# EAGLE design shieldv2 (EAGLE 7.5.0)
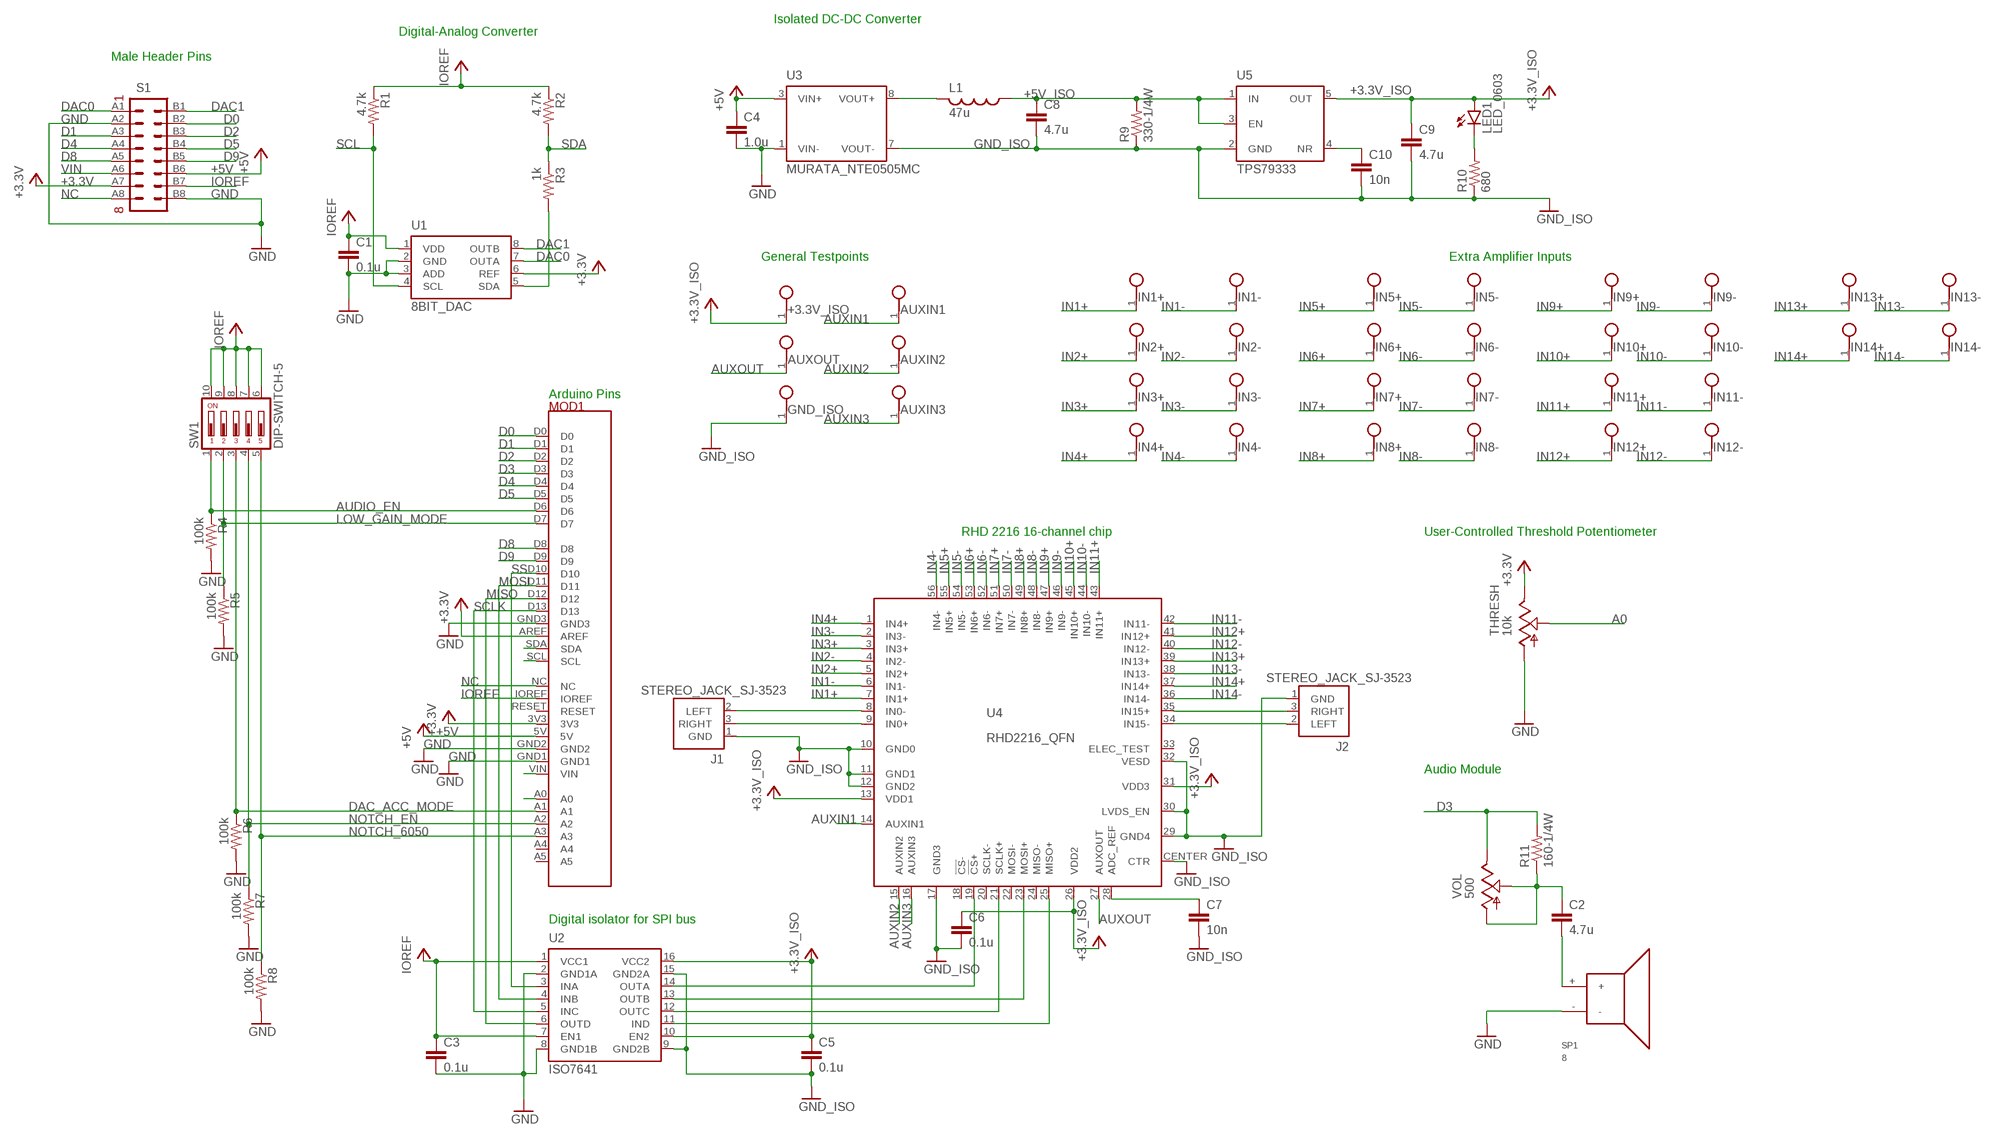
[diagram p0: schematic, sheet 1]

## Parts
+3.3V_ISO  TESTPOINT  [TESTPOINT]
AUXIN1  TESTPOINT  [TESTPOINT]
AUXIN2  TESTPOINT  [TESTPOINT]
AUXIN3  TESTPOINT  [TESTPOINT]
AUXOUT  TESTPOINT  [TESTPOINT]
C1  0.1u  C_0603  [0603]
C2  4.7u  C_0805  [0805]
C3  0.1u  C_0603  [0603]
C4  1.0u  C_0805  [0805]
C5  0.1u  C_0603  [0603]
C6  0.1u  C_0603  [0603]
C7  10n  C_0603  [0603]
C8  4.7u  C_0805  [0805]
C9  4.7u  C_0805  [0805]
C10  10n  C_0603  [0603]
GND_ISO  TESTPOINT  [TESTPOINT]
IN1+  TESTPOINT  [TESTPOINT]
IN1-  TESTPOINT  [TESTPOINT]
IN2+  TESTPOINT  [TESTPOINT]
IN2-  TESTPOINT  [TESTPOINT]
IN3+  TESTPOINT  [TESTPOINT]
IN3-  TESTPOINT  [TESTPOINT]
IN4+  TESTPOINT  [TESTPOINT]
IN4-  TESTPOINT  [TESTPOINT]
IN5+  TESTPOINT  [TESTPOINT]
IN5-  TESTPOINT  [TESTPOINT]
IN6+  TESTPOINT  [TESTPOINT]
IN6-  TESTPOINT  [TESTPOINT]
IN7+  TESTPOINT  [TESTPOINT]
IN7-  TESTPOINT  [TESTPOINT]
IN8+  TESTPOINT  [TESTPOINT]
IN8-  TESTPOINT  [TESTPOINT]
IN9+  TESTPOINT  [TESTPOINT]
IN9-  TESTPOINT  [TESTPOINT]
IN10+  TESTPOINT  [TESTPOINT]
IN10-  TESTPOINT  [TESTPOINT]
IN11+  TESTPOINT  [TESTPOINT]
IN11-  TESTPOINT  [TESTPOINT]
IN12+  TESTPOINT  [TESTPOINT]
IN12-  TESTPOINT  [TESTPOINT]
IN13+  TESTPOINT  [TESTPOINT]
IN13-  TESTPOINT  [TESTPOINT]
IN14+  TESTPOINT  [TESTPOINT]
IN14-  TESTPOINT  [TESTPOINT]
J1  STEREO_JACK_SJ-3523  [SJ-3523]
J2  STEREO_JACK_SJ-3523  [SJ-3523]
L1  47u  L_1210  [1210]
LED1  LED_0603  [0603_DIODE]
MOD1  UNOHEADERS  [UNOHEADERS]
R1  4.7k  R_0603  [0603]
R2  4.7k  R_0603  [0603]
R3  1k  R_0603  [0603]
R4  100k  R_0603  [0603]
R5  100k  R_0603  [0603]
R6  100k  R_0603  [0603]
R7  100k  R_0603  [0603]
R8  100k  R_0603  [0603]
R9  330-1/4W  R_0603  [0603]
R10  680  R_0603  [0603]
R11  160-1/4W  R_0603  [0603]
S1  100MIL_HEADER_8X2  [100MIL_HEADER_8X2]
SP1  8  PCM_SPEAKER  [PCM_SPEAKER]
SW1  DIP-SWITCH-5  [DIP-SWITCH-5]
THRESH  10k  POT_SLIDE  [SLIDE_POT_REPLACEMENT]
U1  8BIT_DAC  [UMAX]
U2  ISO7641  [SOIC-16-WIDE]
U3  MURATA_NTE0505MC  [MURATA_NTE]
U4  RHD2216_QFN  [QFN56_8_X_8_LARGE]
U5  TPS79333  [SOT-23-5]
VOL  500  POT_ROT  [ROT_POT_REPLACEMENT]

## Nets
+3.3V: MOD1.3V3 MOD1.AREF S1.A7 THRESH.3 U1.6(REF)
+3.3V_ISO [power]: +3.3V_ISO.1 C5.1 C6.1 C9.1 LED1.A U2.10(EN2) U2.16(VCC2) U4.13(VDD1) U4.26(VDD2) U4.31(VDD3) U5.5(OUT)
+5V: C4.1 MOD1.5V S1.B6 U3.3(VIN+)
+5V_ISO [power]: C8.1 L1.1 R9.2 U5.1(IN) U5.3(EN)
A0: MOD1.A0 THRESH.2
AUDIO_EN: MOD1.D6 R4.1 SW1.1
AUXIN1: AUXIN1.1 U4.14(AUXIN1)
AUXIN2: AUXIN2.1 U4.15(AUXIN2)
AUXIN3: AUXIN3.1 U4.16(AUXIN3)
AUXOUT: AUXOUT.1 U4.27(AUXOUT)
D0: MOD1.D0 S1.B2
D1: MOD1.D1 S1.A3
D2: MOD1.D2 S1.B3
D3: MOD1.D3 R11.2 VOL.3
D4: MOD1.D4 S1.A4
D5: MOD1.D5 S1.B4
D8: MOD1.D8 S1.A5
D9: MOD1.D9 S1.B5
DAC0: S1.A1 U1.7(OUTA)
DAC1: S1.B1 U1.8(OUTB)
DAC_ACC_MODE: MOD1.A1 R6.1 SW1.3
GND: C1.2 C3.2 C4.2 MOD1.GND1 MOD1.GND2 MOD1.GND3 R4.2 R5.2 R6.2 R7.2 R8.2 S1.A2 S1.B8 SP1.- THRESH.1 U1.2(GND) U1.3(ADD) U2.2(GND1A) U2.8(GND1B) U3.1(VIN-)
GND_ISO: C5.2 C6.2 C7.2 C8.2 C9.2 C10.2 GND_ISO.1 J1.1(GND) J2.1(GND) R9.1 R10.1 U2.9(GND2B) U2.15(GND2A) U3.7(VOUT-) U4.10(GND0) U4.11(GND1) U4.12(GND2) U4.17(GND3) U4.29(GND4) U4.30(LVDS_EN) U4.32(VESD) U4.CENTER(CTR) U5.2(GND)
IN1+ [power]: IN1+.1 U4.7(IN1+)
IN1-: IN1-.1 U4.6(IN1-)
IN2+: IN2+.1 U4.5(IN2+)
IN2-: IN2-.1 U4.4(IN2-)
IN3+: IN3+.1 U4.3(IN3+)
IN3-: IN3-.1 U4.2(IN3-)
IN4+: IN4+.1 U4.1(IN4+)
IN4-: IN4-.1 U4.56(IN4-)
IN5+ [power]: IN5+.1 U4.55(IN5+)
IN5-: IN5-.1 U4.54(IN5-)
IN6+ [power]: IN6+.1 U4.53(IN6+)
IN6-: IN6-.1 U4.52(IN6-)
IN7+: IN7+.1 U4.51(IN7+)
IN7-: IN7-.1 U4.50(IN7-)
IN8+: IN8+.1 U4.49(IN8+)
IN8-: IN8-.1 U4.48(IN8-)
IN9+: IN9+.1 U4.47(IN9+)
IN9-: IN9-.1 U4.46(IN9-)
IN10+ [power]: IN10+.1 U4.45(IN10+)
IN10-: IN10-.1 U4.44(IN10-)
IN11+: IN11+.1 U4.43(IN11+)
IN11-: IN11-.1 U4.42(IN11-)
IN12+: IN12+.1 U4.41(IN12+)
IN12-: IN12-.1 U4.40(IN12-)
IN13+: IN13+.1 U4.39(IN13+)
IN13-: IN13-.1 U4.38(IN13-)
IN14+: IN14+.1 U4.37(IN14+)
IN14-: IN14-.1 U4.36(IN14-)
IOREF: C1.1 C3.1 MOD1.IOREF R1.1 R2.1 S1.B7 SW1.6 SW1.7 SW1.8 SW1.9 SW1.10 U1.1(VDD) U2.1(VCC1) U2.7(EN1)
LOW_GAIN_MODE: MOD1.D7 R5.1 SW1.2
MISO: MOD1.D12 U2.6(OUTD)
MOSI: MOD1.D11 U2.4(INB)
N$1: U2.14(OUTA) U4.19(!CS!+)
N$2: C2.1 R11.1 VOL.1 VOL.2
N$3: C2.2 SP1.+
N$4: U2.13(OUTB) U4.23(MOSI+)
N$6: U2.12(OUTC) U4.21(SCLK+)
N$7: U2.11(IND) U4.25(MISO+)
N$11: L1.2 U3.8(VOUT+)
N$12: LED1.C R10.2
N$13: C7.1 U4.28(ADC_REF)
N$14: C10.1 U5.4(NR)
N$18: J1.2(LEFT) U4.8(IN0-)
N$19: J1.3(RIGHT) U4.9(IN0+)
N$30: J2.3(RIGHT) U4.35(IN15+)
N$31: J2.2(LEFT) U4.34(IN15-)
NC: MOD1.NC S1.A8
NOTCH_6050: MOD1.A3 R8.1 SW1.5
NOTCH_EN: MOD1.A2 R7.1 SW1.4
PRESDA: R3.2 U1.5(SDA)
SCL: MOD1.SCL R1.2 U1.4(SCL)
SCLK: MOD1.D13 U2.5(INC)
SDA: MOD1.SDA R2.2 R3.1
SS: MOD1.D10 U2.3(INA)
VIN: MOD1.VIN S1.A6
Unconnected: MOD1.A4 MOD1.A5 MOD1.RESET U4.18(!CS!-) U4.20(SCLK-) U4.22(MOSI-) U4.24(MISO-) U4.33(ELEC_TEST)

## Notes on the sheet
- Isolated DC-DC Converter
- Digital-Analog Converter
- Male Header Pins
- General Testpoints | Extra Amplifier Inputs
- Arduino Pins
- RHD 2216 16-channel chip | User-Controlled Threshold Potentiometer
- Audio Module
- Digital isolator for SPI bus

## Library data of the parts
+3.3V_ISO AUXIN1-AUXIN3 AUXOUT GND_ISO IN1+ IN1- IN2+ IN2- IN3+ IN3- IN4+ IN4- IN5+ IN5- IN6+ IN6- IN7+ IN7- IN8+ IN8- IN9+ IN9- IN10+ IN10- IN11+ IN11- IN12+ IN12- IN13+ IN13- IN14+ IN14- = RHD2000_eval_board:TESTPOINT: PCB Test Point
C1-C10 = CLAMP_interface_board:C: Capacitor
J1 J2 = CLAMP_interface_board:STEREO_JACK: CUI Inc. SJ-3523 stereo audio jack
L1 = CLAMP_interface_board:L: Inductor
LED1 = CLAMP_interface_board:LED
MOD1 = intan-arduino:UNOHEADERS: Headers for connecting an Arduino UNO to a shield
R1-R11 = CLAMP_interface_board:R: Resistor
S1 = intan-arduino:100MIL_HEADER_8X2: 8 rows of 2 header pins, 100 mil spacing. DigiKey: 609-3486-1-ND
SP1 = intan-arduino:PCM_SPEAKER
SW1 = intan-arduino:DIP-SWITCH-5
THRESH VOL = intan-arduinov2:POT: Potentiometer
U1 = intan-arduino:8BIT_DAC: 8-bit 2 Wire Serial DAC. Digikey Part Number MAX5820LEUA+-ND
U2 = CLAMP_interface_board:ISO7641: TI ISO7641FM Quad-Channel Digital Isolator
U3 = CLAMP_interface_board:MURATA_NTE0505MC: Murata NTE0505MC Isolated 1W +5V to +5V DC/DC Converter
U4 = harrison:RHD2216
U5 = CLAMP_interface_board:TPS79333: Texas Instruments TPS79333 3.3V LDO regulator

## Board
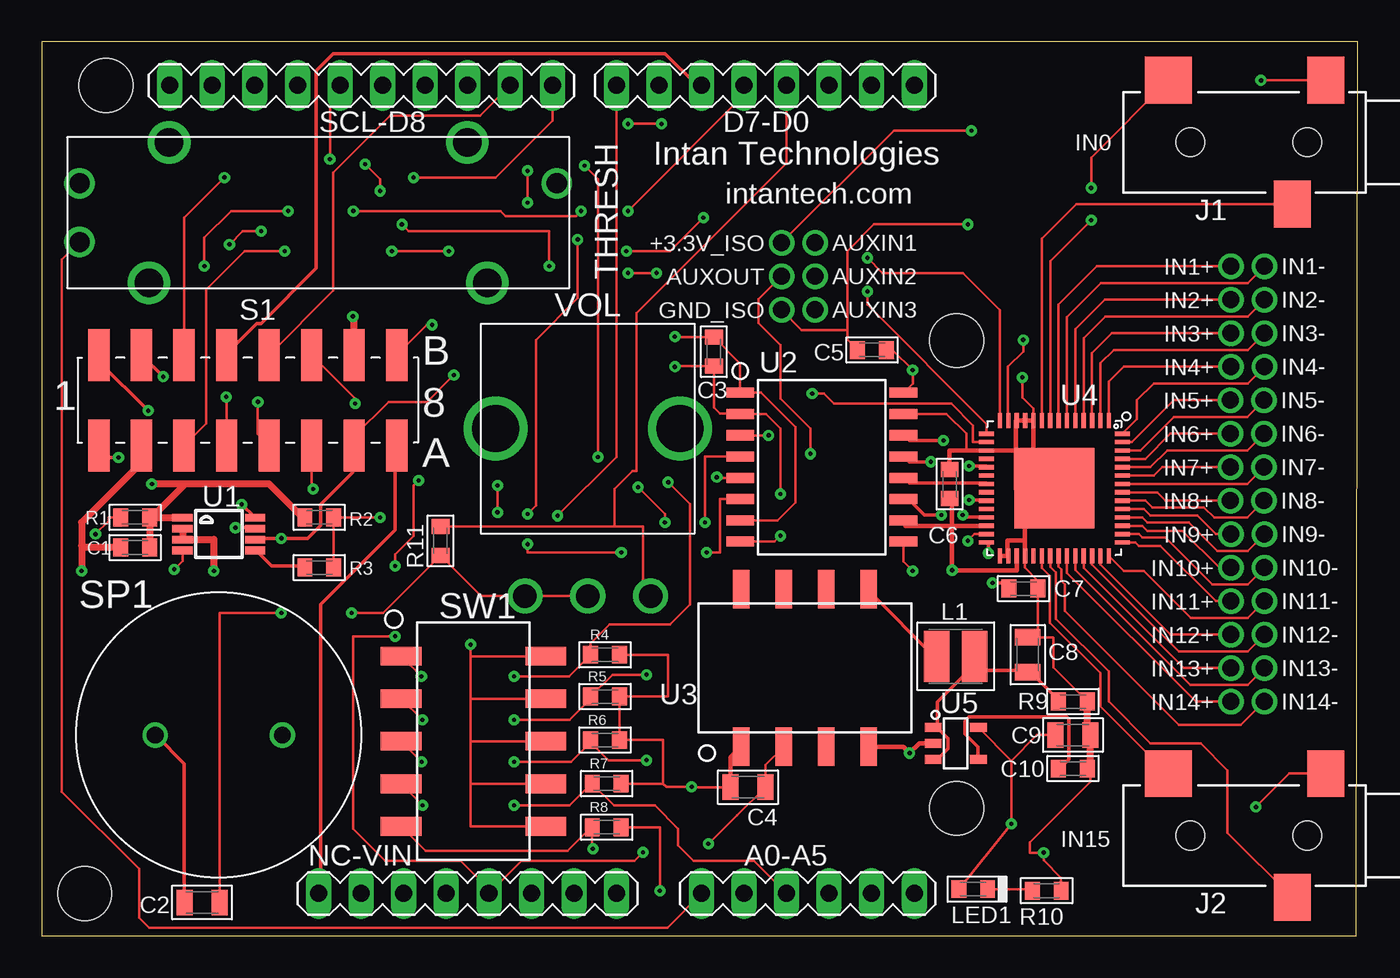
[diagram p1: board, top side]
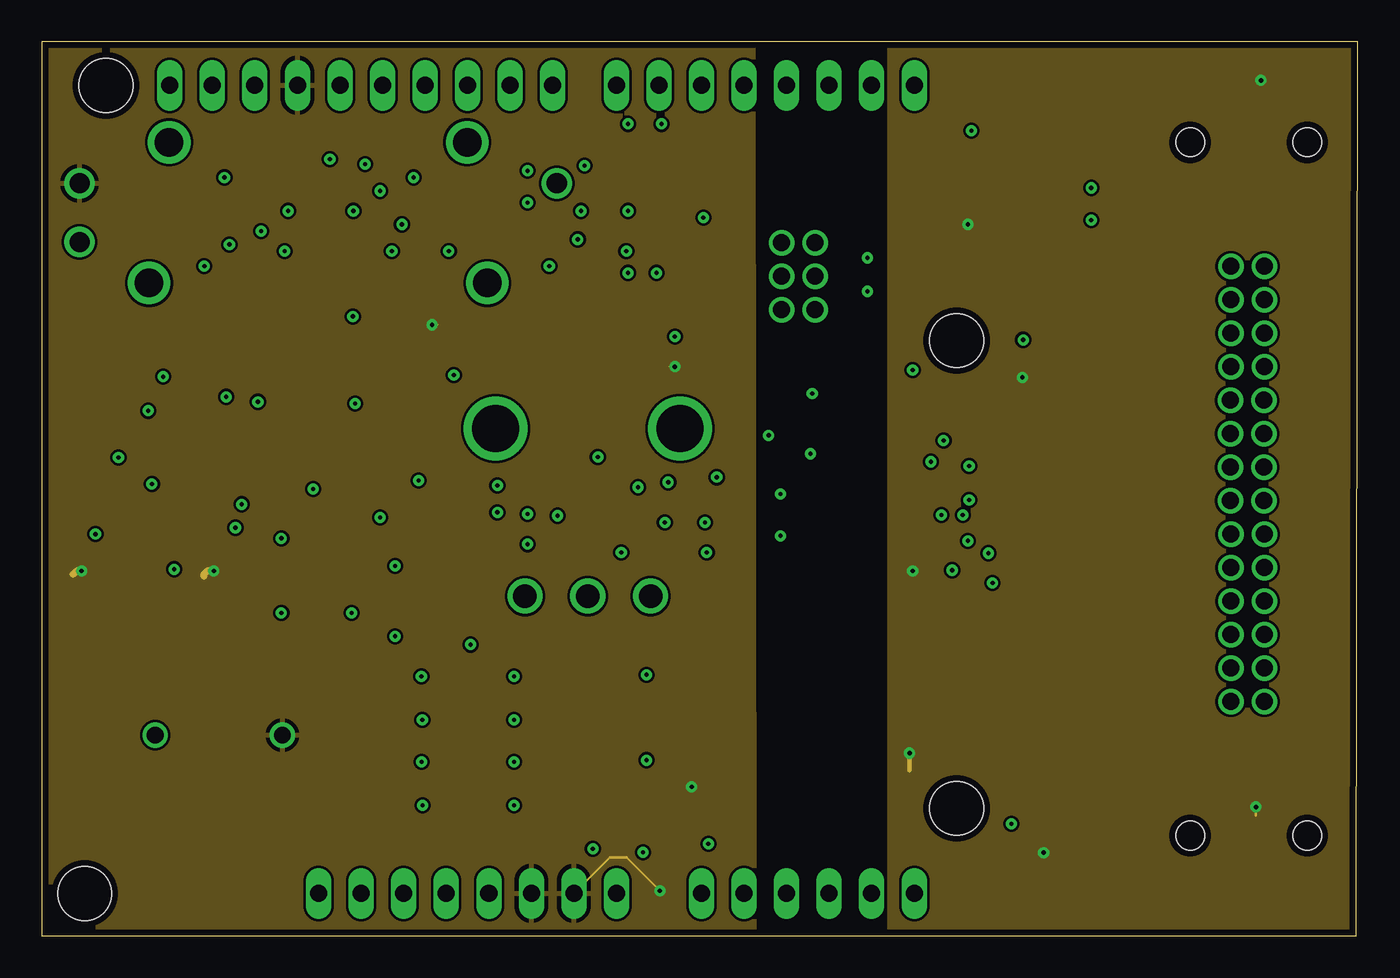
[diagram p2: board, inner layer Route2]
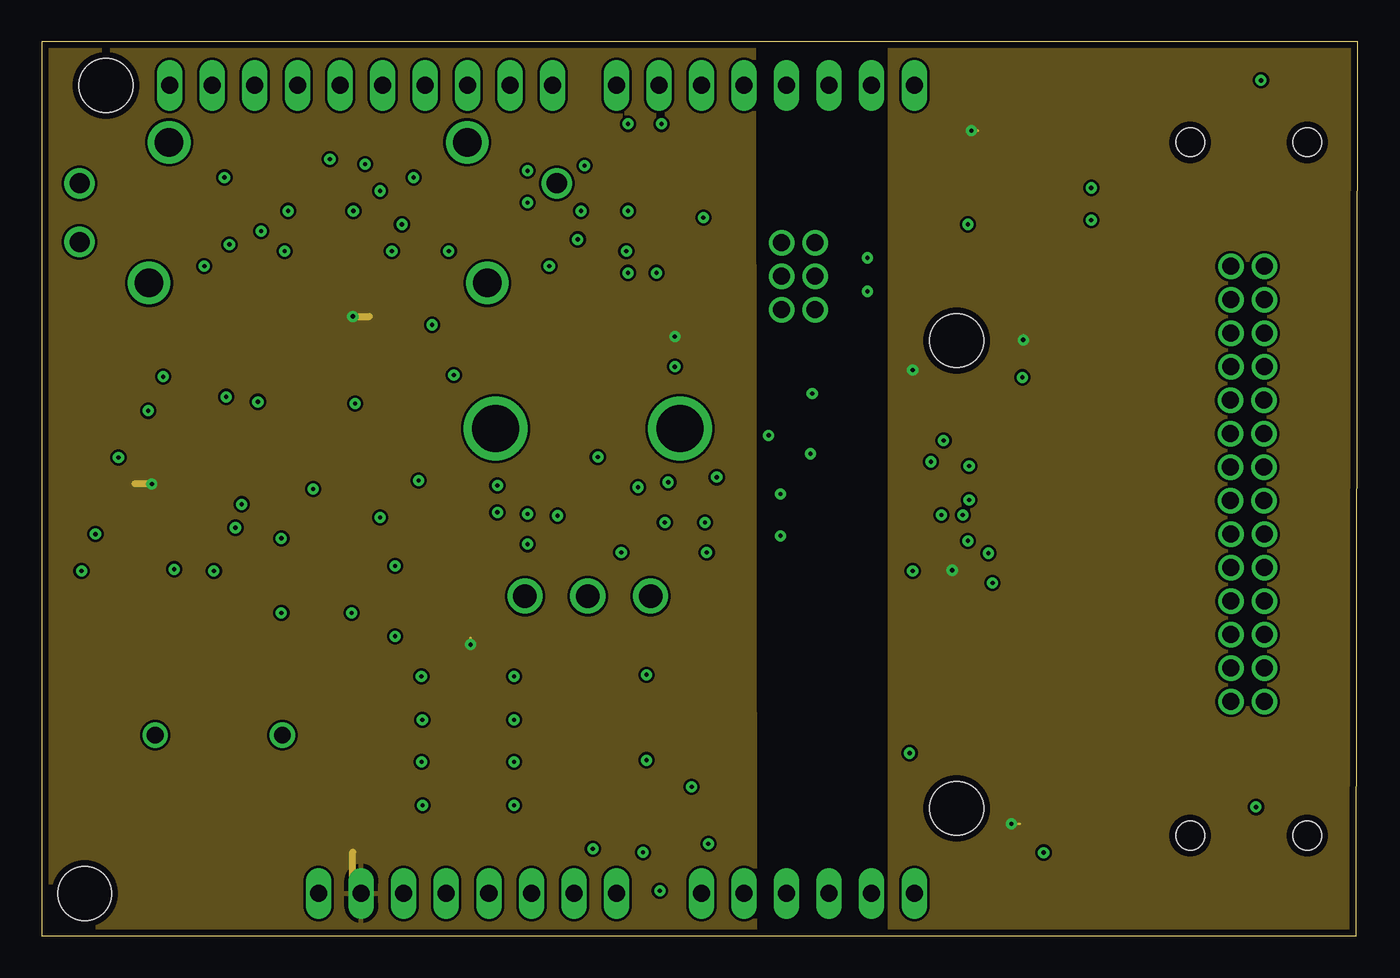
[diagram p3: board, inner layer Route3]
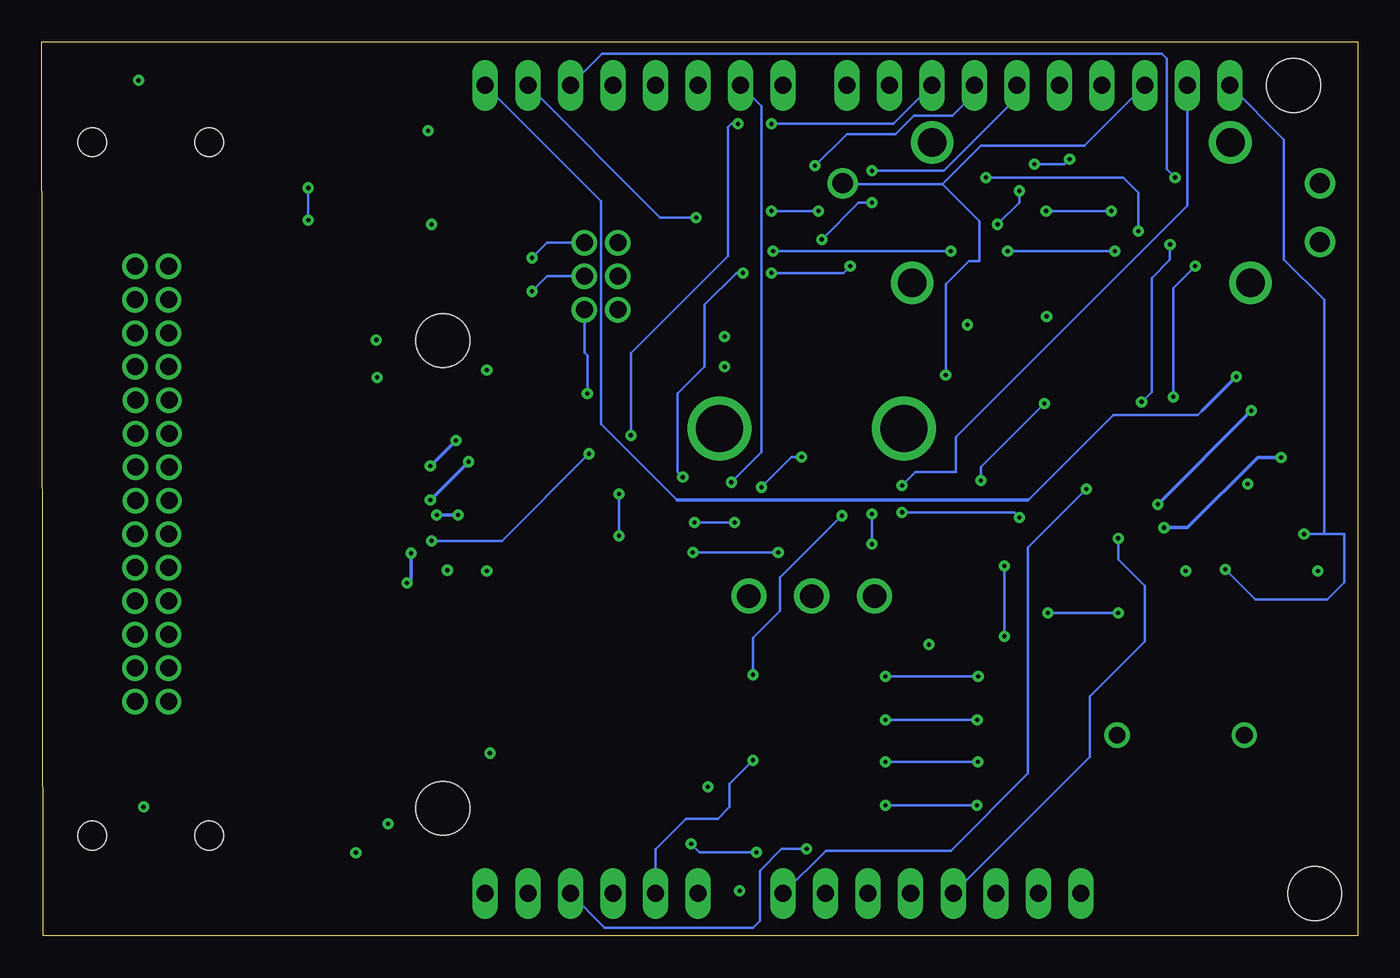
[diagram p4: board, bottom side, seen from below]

Size 78.57 x 53.4 mm. Coordinates in mm from the lower left corner, seen from the top.
Outline: 0,0 78.5,0 78.57,53.4 0,53.4 0,0
Copper layers (1*2+3*16): Top 0.035mm / dielectric 1.5mm / Route2 0.035mm / dielectric 0.15mm / Route3 0.035mm / dielectric 0.2mm / Bottom 0.035mm
Design rules "default *": minimum track width 6mil, minimum drill 10mil, track to track 6mil, track to pad 6mil, pad to pad 6mil, via to via 6mil, smd to smd 6mil, copper to edge 15mil, drill to drill 8mil, minimum pad ring 10mil, minimum via ring 8mil, stop-mask expansion 4mil, vias tented up to drill 0mil, thermal gap 10mil

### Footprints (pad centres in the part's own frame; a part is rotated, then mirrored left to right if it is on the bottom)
TESTPOINT = drill 1.016: 1 0,0
0603 = smd 0.889 x 1.067: 1 -0.864,0; 2 0.864,0
0805 = smd 0.965 x 1.524: 1 -1.041,0; 2 1.041,0
SJ-3523 = smd 2.2 x 2.8: 1 -1.1,-3.7; 3 0.9,3.7 | smd 2.8 x 2.8: 2 8.3,-3.7 | hole 1.7: 7,0; 0,0
1210 = smd 1.524 x 3.048: 1 -1.143,0; 2 1.143,0
0603_DIODE = smd 0.889 x 1.067: A 0.864,0; C -0.864,0
UNOHEADERS = drill 1.016 long: 3V3 -29.21,-49.53; 5V -26.67,-49.53; A0 -13.97,-49.53; A1 -11.43,-49.53; A2 -8.89,-49.53; A3 -6.35,-49.53; A4 -3.81,-49.53; A5 -1.27,-49.53; AREF -40.64,-1.27; D0 -1.27,-1.27; D1 -3.81,-1.27; D2 -6.35,-1.27; D3 -8.89,-1.27; D4 -11.43,-1.27; D5 -13.97,-1.27; D6 -16.51,-1.27; D7 -19.05,-1.27; D8 -22.86,-1.27; D9 -25.4,-1.27; D10 -27.94,-1.27; D11 -30.48,-1.27; D12 -33.02,-1.27; D13 -35.56,-1.27; GND1 -21.59,-49.53; GND2 -24.13,-49.53; GND3 -38.1,-1.27; IOREF -34.29,-49.53; NC -36.83,-49.53; RESET -31.75,-49.53; SCL -45.72,-1.27; SDA -43.18,-1.27; VIN -19.05,-49.53 | hole 3.2: -49.53,-1.27; 1.27,-16.51; 1.27,-44.45; -50.8,-49.53
100MIL_HEADER_8X2 = smd 1.27 x 3.1: A1 -10.16,-2.7; A2 -7.62,-2.7; A3 -5.08,-2.7; A4 -2.54,-2.7; A5 0,-2.7; A6 2.54,-2.7; A7 5.08,-2.7; A8 7.62,-2.7; B1 -10.16,2.7; B2 -7.62,2.7; B3 -5.08,2.7; B4 -2.54,2.7; B5 0,2.7; B6 2.54,2.7; B7 5.08,2.7; B8 7.62,2.7
PCM_SPEAKER = drill 1: + -3.8,0; - 3.8,0
DIP-SWITCH-5 = smd 1.118 x 2.438: 1 -3.81,-4.318; 2 -1.27,-4.318; 3 1.27,-4.318; 4 3.81,-4.318; 5 6.35,-4.318; 6 6.35,4.318; 7 3.81,4.318; 8 1.27,4.318; 9 -1.27,4.318; 10 -3.81,4.318
SLIDE_POT_REPLACEMENT = drill 1.2: 1 -14.25,1.75; 2 -14.25,-1.75; 3 14.25,1.75 | drill 1.7: H1 -10.1,-4.2; H2 10.1,-4.2; H3 8.9,4.2; H4 -8.9,4.2
UMAX = smd 0.45 x 1.2: 1 -0.975,-2.175; 2 -0.325,-2.175; 3 0.325,-2.175; 4 0.975,-2.175; 5 0.975,2.175; 6 0.325,2.175; 7 -0.325,2.175; 8 -0.975,2.175
SOIC-16-WIDE = smd 0.6 x 1.65: 1 -4.445,-4.875; 2 -3.175,-4.875; 3 -1.905,-4.875; 4 -0.635,-4.875; 5 0.635,-4.875; 6 1.905,-4.875; 7 3.175,-4.875; 8 4.445,-4.875; 9 4.445,4.875; 10 3.175,4.875; 11 1.905,4.875; 12 0.635,4.875; 13 -0.635,4.875; 14 -1.905,4.875; 15 -3.175,4.875; 16 -4.445,4.875
MURATA_NTE = smd 1 x 2.3: 1 -3.81,-4.7; 3 -1.27,-4.7; 5 1.27,-4.7; 7 3.81,-4.7; 8 3.81,4.7; 10 1.27,4.7; 12 -1.27,4.7; 14 -3.81,4.7
QFN56_8_X_8_LARGE = smd 0.9 x 0.25: 1 -4.05,3.25; 2 -4.05,2.75; 3 -4.05,2.25; 4 -4.05,1.75; 5 -4.05,1.25; 6 -4.05,0.75; 7 -4.05,0.25; 8 -4.05,-0.25; 9 -4.05,-0.75; 10 -4.05,-1.25; 11 -4.05,-1.75; 12 -4.05,-2.25; 13 -4.05,-2.75; 14 -4.05,-3.25; 29 4.05,-3.25; 30 4.05,-2.75; 31 4.05,-2.25; 32 4.05,-1.75; 33 4.05,-1.25; 34 4.05,-0.75; 35 4.05,-0.25; 36 4.05,0.25; 37 4.05,0.75; 38 4.05,1.25; 39 4.05,1.75; 40 4.05,2.25; 41 4.05,2.75; 42 4.05,3.25 | smd 0.25 x 0.9: 15 -3.25,-4.05; 16 -2.75,-4.05; 17 -2.25,-4.05; 18 -1.75,-4.05; 19 -1.25,-4.05; 20 -0.75,-4.05; 21 -0.25,-4.05; 22 0.25,-4.05; 23 0.75,-4.05; 24 1.25,-4.05; 25 1.75,-4.05; 26 2.25,-4.05; 27 2.75,-4.05; 28 3.25,-4.05; 43 3.25,4.05; 44 2.75,4.05; 45 2.25,4.05; 46 1.75,4.05; 47 1.25,4.05; 48 0.75,4.05; 49 0.25,4.05; 50 -0.25,4.05; 51 -0.75,4.05; 52 -1.25,4.05; 53 -1.75,4.05; 54 -2.25,4.05; 55 -2.75,4.05; 56 -3.25,4.05 | smd 4.8 x 4.8: CENTER 0,0
SOT-23-5 = smd 0.55 x 1: 1 -0.95,-1.35; 2 0,-1.35; 3 0.95,-1.35; 4 0.95,1.35; 5 -0.95,1.35
ROT_POT_REPLACEMENT = drill 1.4: 1 -3.75,-10; 2 0,-10; 3 3.75,-10 | drill 2.8: H1 -5.5,0; H2 5.5,0

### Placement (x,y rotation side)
+3.3V_ISO  44.17,41.4 180 top
AUXIN1  46.17,41.4 0 top
AUXIN2  46.17,39.4 0 top
AUXIN3  46.17,37.4 0 top
AUXOUT  44.17,39.4 180 top
C1  5.57,23.2 180 top
C2  9.57,2 180 top
C3  40.13,34.9 270 top
C4  42.16,8.89 180 top
C5  49.57,35 180 top
C6  54.21,26.98 90 top
C7  58.62,20.75 0 top
C8  58.87,16.8 90 top
C9  61.57,12 0 top
C10  61.57,10 0 top
GND_ISO  44.17,37.4 180 top
IN1+  71,40 180 top
IN1-  73,40 0 top
IN2+  71,38 180 top
IN2-  73,38 0 top
IN3+  71,36 180 top
IN3-  73,36 0 top
IN4+  71,34 180 top
IN4-  73,34 0 top
IN5+  70.97,32 180 top
IN5-  72.97,32 0 top
IN6+  70.97,30 180 top
IN6-  72.97,30 0 top
IN7+  70.97,28 180 top
IN7-  72.97,28 0 top
IN8+  70.97,26 180 top
IN8-  72.97,26 0 top
IN9+  71,24 180 top
IN9-  73,24 0 top
IN10+  71,22 180 top
IN10-  73,22 0 top
IN11+  71,20 180 top
IN11-  73,20 0 top
IN12+  71,18 180 top
IN12-  73,18 0 top
IN13+  71,16 180 top
IN13-  73,16 0 top
IN14+  71,14 180 top
IN14-  73,14 0 top
J1  75.57,47.4 180 top
J2  75.57,6 180 top
L1  54.57,16.7 180 top
LED1  55.61,2.8 180 top
MOD1  53.36,52.07 0 top
R1  5.57,25 180 top
R2  16.57,25 0 top
R3  16.57,22 180 top
R4  33.63,16.8 0 top
R5  33.63,14.3 0 top
R6  33.63,11.7 0 top
R7  33.73,9.1 0 top
R8  33.73,6.5 0 top
R9  61.57,14 180 top
R10  60,2.7 180 top
R11  23.8,23.6 90 top
S1  13.57,32 0 top
SP1  10.57,12 0 top
SW1  25.77,12.9 270 top
THRESH  16.5,43.2 0 top
U1  10.57,24 270 top
U2  46.57,28 270 top
U3  45.57,16 0 top
U4  60.46,26.75 270 top
U5  54.57,11.5 270 top
VOL  32.6,30.3 0 top

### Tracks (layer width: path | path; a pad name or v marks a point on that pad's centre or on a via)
+3.3V  (via drill 0.25)
  Top 0.152: v24.6,33.5 23,31.9 20.7,31.9 18.65,29.85 S1.A7
  Top 0.203: U1.6 12.83,23.75 v14.3,23.75 15.88,23.75 16.64,24.51 16.64,25.78 18.54,27.69 18.54,29.21 S1.A7
  Bottom 0.152: v24.6,33.5 24.6,38.92 23.22,40.3 22.6,40.3 22.6,42.7 24.8,44.9 | MOD1.3V3 16,10.69 16,14.3 12.7,17.6 12.7,20.9 14.3,22.5 v14.3,23.75 | MOD1.AREF 16.32,47.2 22.5,47.2 24.8,44.9 | 24.8,44.9 30.7,44.9 THRESH.3
+3.3V_ISO  (via drill 0.25)
  Top 0.152: U5.5 57.9,10.47 | 57.9,10.47 v57.9,6.7 LED1.A | 57.9,10.47 59.43,12 C9.1 | +3.3V_ISO.1 50.87,48.1 v55.5,48.1 | U4.13 57.7,34 58.6,34.9 v58.6,35.6 | C5.1 50.8,35 v52,33.8 52,33 U2.16
  Top 0.254: U4.31 58.21,21.84 v54.36,21.84 54.36,24.5 | U2.10 51.45,24.89 51.56,24.89 51.56,24.5 54.36,24.5 | U4.26 54.36,24.5 | 54.36,24.5 54.36,25.97 C6.1
  Route3 0.152: v57.9,6.7 58.4,6.7 | v55.5,48.1 55.9,48.1 | v58.6,35.6 58.6,35.9 | v52,33.8 52.2,33.8
  pour Route3: 50.65,0 78.5,0 78.5,53.5 50.65,53.5
+5V  (via drill 0.25)
  Top 0.152: v35.9,5 35.4,4.5 28.65,4.5 MOD1.5V 26.69,2.81 25,4.5 20.5,4.5 18.6,6.4 18.6,17.9 v21.1,17.9 | v39.8,5.5 41.5,7.2 41.52,7.2 C4.1 43.2,10.21 U3.3 | S1.B6 18.7,32.11 v18.7,31.8 | v22.5,27.2 22.2,26.9 22.2,23.9 21.1,22.8 v21.1,22.1
  Bottom 0.152: v35.9,5 39.3,5 v39.8,5.5 | v18.7,31.8 22.5,28 v22.5,27.2 | v21.1,22.1 v21.1,17.9
+5V_ISO
  Top 0.203: R9.2 60.71,14.1 58.93,15.88 C8.1 58.8,15.88 55.5,15.88 L1.1 55.63,16.64 55.63,16.13 53.47,13.97 53.47,12.57 U5.1 53.34,12.57 54.1,11.81 54.1,11.18 53.59,10.67 53.34,10.67 U5.3
A0
  Top 0.152: THRESH.2 1.2,40.4 1.2,8.6 5.8,4 5.8,1.1 6.4,0.5 37.35,0.5 MOD1.A0
AUDIO_EN  (via drill 0.25)
  Top 0.152: SW1.1 v22.66,15.5 | v28.2,15.5 31.47,15.5 R4.1 32.77,17.47 33.9,18.6 37.5,18.6 38.7,19.8 38.7,25.8 v37.4,27.1
  Bottom 0.152: v28.2,15.5 v22.66,15.5 | v37.4,27.1 35.6,28.9 35.6,49.55 MOD1.D6
AUXIN1  (via drill 0.25)
  Top 0.152: U4.14 57.21,37.39 55,39.6 50.2,39.6 v49.3,40.5
  Bottom 0.152: AUXIN1.1 48.4,41.4 v49.3,40.5
AUXIN2  (via drill 0.25)
  Top 0.152: U4.15 56.41,30.59 49.3,37.7 v49.3,38.5
  Bottom 0.152: AUXIN2.1 48.4,39.4 v49.3,38.5
AUXIN3  (via drill 0.25)
  Top 0.152: U4.16 55.6,29.5 55.6,30.5 54.3,31.8 47.3,31.8 46.7,32.4 v46,32.4
  Bottom 0.152: AUXIN3.1 46.17,34.83 46,34.66 v46,32.4
AUXOUT  (via drill 0.25)
  Top 0.152: U4.27 55.7,24 v55.3,23.6 | AUXOUT.1 42.8,38.03 42.8,36.6 44.1,35.3 44.1,32.1 45.9,30.3 v45.9,28.8
  Bottom 0.152: v55.3,23.6 51.1,23.6 v45.9,28.8
D0  (via drill 0.25)
  Top 0.203: v7.24,33.4 5.97,34.67 S1.B2
  Bottom 0.152: 9.27,31.37 9.54,31.1 14.6,31.1 19.66,26.04 19.68,26.04 | 40.64,26.04 45.17,30.57 45.17,43.88 MOD1.D0
  Bottom 0.203: 19.68,26.04 40.64,26.04 | v7.24,33.4 9.27,31.37 | 52.07,50.8 MOD1.D0
D1  (via drill 0.25)
  Top 0.152: S1.A3 9.8,30.61 9.8,38.6 12.1,40.9 v14.5,40.9 | v34.9,40.9 37.5,40.9 v39.5,42.9 | v20.9,40.9 v24.3,40.9
  Bottom 0.152: v39.5,42.9 41.65,42.9 MOD1.D1 | v14.5,40.9 v20.9,40.9 | v24.3,40.9 v34.9,40.9
D2  (via drill 0.25)
  Top 0.152: S1.B3 8.49,42.89 v10.9,45.3
  Bottom 0.152: v10.9,45.3 11.4,45.8 11.4,52.4 11.7,52.7 45.11,52.7 MOD1.D2
D3
  Top 0.152: R11.2 34.2,24.46 | 34.2,24.46 35.9,24.46 35.9,20.75 VOL.3 | MOD1.D3 44.47,46.17 35.5,37.2 35.5,27.78 35.28,27.78 34.2,26.7 34.2,24.46
D4  (via drill 0.25)
  Top 0.152: S1.A4 11.03,32.17 v11,32.2 | v9.7,40 9.7,41.7 11.3,43.3 v14.7,43.3 | v35,43.3 41.93,50.23 MOD1.D4 | v32.2,43.3 31.9,43 27.7,43 27.4,43.3 v18.6,43.3
  Bottom 0.152: v11,32.2 11,38.7 v9.7,40 | v14.7,43.3 v18.6,43.3 | v32.2,43.3 v35,43.3
D5
  Top 0.203: MOD1.D5 39.12,50.8 37.21,52.7 17.4,52.7 16.38,51.69 16.38,39.88 13.08,36.58 12.83,36.58 11.05,34.8 S1.B4
D8  (via drill 0.25)
  Top 0.152: S1.A5 12.9,29.97 v12.9,31.9 | v11.2,41.3 12,42.1 v13.1,42.1 | v22.2,45.3 27.1,45.3 30.5,48.7 MOD1.D8
  Bottom 0.152: v12.9,31.9 12.3,32.5 12.3,39.3 11.2,40.4 v11.2,41.3 | v13.1,42.1 13.1,44.4 14,45.3 v22.2,45.3
D9
  Top 0.152: S1.B5 17.4,38.53 17.4,45.6 20.8,49 26.16,49 MOD1.D9
DAC0  (via drill 0.25)
  Top 0.203: v11.56,24.38 12.7,24.38 U1.7 | v4.57,28.57 4.06,28.57 3.43,29.21 S1.A1
  Bottom 0.203: v11.56,24.38 10.16,24.38 5.97,28.57 v4.57,28.57
DAC1  (via drill 0.25)
  Top 0.203: 3.3,34.67 S1.B1 3.43,34.67 3.43,34.29 v6.35,31.37 | v11.94,25.78 12.7,25.02 U1.8
  Bottom 0.203: v6.35,31.37 v11.94,25.78
DAC_ACC_MODE  (via drill 0.25)
  Top 0.152: SW1.3 v22.68,10.4 | 32.77,11.57 31.6,10.4 v28.2,10.4 | 32.77,11.57 R6.1 | 32.77,11.57 33.83,10.5 v36.1,10.5
  Bottom 0.152: v28.2,10.4 v22.68,10.4 | v36.1,10.5 37.5,9.1 37.5,7.7 38.2,7 40.1,7 41.93,5.17 MOD1.A1
GND  (via drill 0.25)
  Top 0.152: 34.49,9.2 R7.2 37.1,9.1 | C4.2 v38.81,8.89 v38.8,8.9 37.3,8.9 37.1,9.1 | v37.8,34 37.84,34.04 C3.2 40.13,31.57 40.5,31.2 41.67,31.2 U2.2 43.23,31.18 44.1,30.3 v44.1,26.4 | v44.1,23.9 43.76,23.55 U2.8 | S1.B8 22.99,36.5 v23.3,36.5 | R4.2 37.4,16.8 37.4,14.3 R5.2 R6.2 37.1,11.7 37.1,9.1 | R8.2 36.9,6.5 v36.9,2.7
  Top 0.254: 41.71,11.25 U3.1 41.12,10.66 C4.2
  Top 0.406: S1.A2 5.95,28.28 2.37,24.7 2.37,23.3 | 2.37,23.3 v2.37,21.8 | C1.2 2.47,23.2 2.37,23.3 | U1.2 U1.3 10.24,23.68 10.27,23.7 v10.27,21.8
  Route2 0.152: v36.9,2.7 34.9,4.7 33.93,4.7 MOD1.GND1 | v38.8,8.9 38.6,8.9 | v37.8,34 37.5,34 | v23.3,36.5 23.6,36.5
  Route2 0.406: v2.37,21.8 2.07,21.8 1.87,21.6 | v10.27,21.8 9.87,21.8 9.67,21.6 9.67,21.5
  Bottom 0.152: v44.1,26.4 v44.1,23.9
  pour Route2: 42.55,0 42.5,53.5 0,53.5 0,0
GND_ISO  (via drill 0.25)
  Top 0.152: 59.48,17.84 C7.2 59.48,21.22 58.7,22 58.7,22.69 U4.32 | C8.2 59.48,17.84 | R9.1 60.4,16.03 60.4,17.8 60.36,17.84 59.48,17.84 | R10.1 60.86,3.46 59.82,4.51 v59.82,4.98 58.99,4.98 58.99,5.59 62.61,9.21 62.61,10 | J2.1 74.5,9.7 v72.5,7.7 | J1.1 v72.8,51.1 | U4.10 59.21,31.51 58.55,32.17 v58.55,33.36 | GND_ISO.1 45.37,36.2 48.1,36.2 | C5.2 48.1,35.61 48.1,36.2 | 48.1,36.2 48.1,40.9 49.7,42.5 v55.3,42.5 | U2.15 54.02,31.18 55.2,30 55.2,29.1 55.3,29 | U2.9 51.45,22.36 v52,21.8
  Top 0.254: U4.29 U4.30 57.66,22.7 57.66,23.62 58.71,23.62 | 58.17,29 58.17,30.8 U4.12 U4.11 U4.10 59.21,28.73 59.18,28.7 | 58.17,29 58.17,26.67 59.69,26.67 | 59.69,26.67 60.46,26.67 U4.CENTER | 58.17,29 U4.17 55.3,29 54.21,29 C6.2 | U5.2 52.39,11.5 v51.82,10.92 51.44,11.3 U3.7 | U4.32 58.71,23.62 | 58.71,23.62 58.71,24.6 58.67,24.64 | 60.21,26.5 U4.CENTER | 62.71,29 U4.CENTER | 59.71,26.65 59.69,26.67 | 62.71,24.5 U4.CENTER
  Top 0.406: C10.2 62.61,10 C9.2 62.43,12 R9.1 62.37,14
  Route2 0.152: v72.5,7.7 72.5,7.2 | v72.8,51.1 72.6,51.1 | v58.55,33.36 58.55,33.54 | v55.3,42.5 55.5,42.5 | v52,21.8 52,21.6 | v59.82,4.98 59.98,4.98
  Route2 0.254: v51.82,10.92 51.82,9.91
  pour Route2: 78.57,0 50.65,0 50.65,53.5 78.57,53.51
IN1+
  Top 0.152: IN1+.1 63.01,40 60.71,37.7 U4.7
IN1-
  Top 0.152: IN1-.1 72,39 63.25,39 61.21,36.97 U4.6
IN2+
  Top 0.152: IN2+.1 63.48,38 61.71,36.23 U4.5
IN2-
  Top 0.152: IN2-.1 72,37 63.5,37 62.21,35.71 U4.4
IN3+
  Top 0.152: IN3+.1 63.9,36 62.71,34.81 U4.3
IN3-
  Top 0.152: IN3-.1 72,35 64,35 63.21,34.21 U4.2
IN4+
  Top 0.152: IN4+.1 64.6,34 63.71,33.11 U4.1
IN4-
  Top 0.152: IN4-.1 72,33 66.4,33 65.4,32 65.4,30.89 U4.56
IN5+
  Top 0.152: IN5+.1 67.6,32 65.1,29.5 U4.55
IN5-
  Top 0.152: IN5-.1 71.97,31 67.6,31 65.6,29 U4.54
IN6+
  Top 0.152: IN6+.1 67.4,30 65.9,28.5 U4.53
IN6-
  Top 0.152: IN6-.1 71.97,29 67.2,29 66.2,28 U4.52
IN7+
  Top 0.152: IN7+.1 66.9,28 66.4,27.5 U4.51
IN7-
  Top 0.152: IN7-.1 71.97,27 69.8,27 U4.50
IN8+
  Top 0.152: IN8+.1 67.1,26 66.6,26.5 U4.49
IN8-
  Top 0.152: IN8-.1 71.97,25 70,25 69.4,25.6 66.3,25.6 65.9,26 U4.48
IN9+
  Top 0.152: IN9+.1 70.1,24 69,25.1 66.2,25.1 65.8,25.5 U4.47
IN9-
  Top 0.152: IN9-.1 72,23 70.2,23 68.5,24.7 66,24.7 65.7,25 U4.46
IN10+
  Top 0.152: IN10+.1 70.3,22 68.1,24.2 66,24.2 65.7,24.5 U4.45
IN10-
  Top 0.152: IN10-.1 72,21 69.9,21 67.1,23.8 65.7,23.8 65.5,24 U4.44
IN11+
  Top 0.152: IN11+.1 70.1,20 66.8,23.3 65.5,23.3 65.3,23.5 U4.43
IN11-
  Top 0.152: IN11-.1 72,19 68.6,19 65.8,21.8 64.61,21.8 U4.42
IN12+
  Top 0.152: IN12+.1 67.4,18 63.21,22.19 U4.41
IN12-
  Top 0.152: IN12-.1 72,17 67.9,17 62.71,22.19 U4.40
IN13+
  Top 0.152: IN13+.1 68.2,16 62.21,21.99 U4.39
IN13-
  Top 0.152: U4.38 61.71,21.86 68.57,15 72,15 IN13-.1
IN14+
  Top 0.152: IN14+.1 68.9,14 61.21,21.69 U4.37
IN14-
  Top 0.152: IN14-.1 71.6,12.6 67.9,12.6 61.1,19.4 61.1,21 60.88,21.22 60.88,21.89 60.71,22.07 U4.36
IOREF  (via drill 0.25)
  Top 0.152: SW1.6 25.6,6.55 25.6,9.09 | 25.6,9.09 25.6,11.63 | 25.6,11.63 25.6,14.17 | 25.6,14.17 25.6,16.71 | SW1.10 25.6,16.71 | 25.6,16.71 v25.6,17.4 | SW1.9 25.6,14.17 | SW1.8 25.6,11.63 | SW1.7 25.6,9.09 | v37.8,35.8 37.8,35.76 C3.1 41.7,34.2 U2.1 42.95,32.45 45,30.4 45,25.9 43.92,24.82 42.83,24.82 42.3,24.82 U2.7
  Top 0.203: U1.1 8.38,25.02 8.37,25
  Top 0.406: R1.1 8.37,25 | R2.1 15.57,25 13.57,27 8.57,27 | 8.57,27 v6.57,27 | R1.1 6.57,25 8.57,27 | S1.B7 18.65,36.92 v18.57,37 | R1.1 C1.1
  Route3 0.152: v25.6,17.4 25.6,17.8 | v37.8,35.8 37.6,35.8
  Route3 0.406: MOD1.IOREF 18.57,2.54 18.57,5 | v6.57,27 5.57,27 | v18.57,37 19.57,37
  pour Route3: 42.55,0 0,0 0,53.5 42.5,53.5
LOW_GAIN_MODE  (via drill 0.25)
  Top 0.152: SW1.2 v22.72,12.9 | v28.2,12.9 31.5,12.9 32.77,14.17 R5.1 34.07,15.6 v36.1,15.6 | v30.8,25.1 34.31,28.61 MOD1.D7
  Bottom 0.152: v28.2,12.9 v22.72,12.9 | v36.1,15.6 36.1,17.8 34.5,19.4 34.5,21.4 v30.8,25.1
MISO  (via drill 0.25)
  Top 0.152: U2.6 40.5,26.09 40.5,22.9 v39.7,22.9 | v34.6,22.9 29,22.9 v29,23.4 | v32,41.6 32,38.1 29.5,35.6 29.5,25.7 v29,25.2 | v29,43.8 v29,45.7
  Bottom 0.152: v39.7,22.9 v34.6,22.9 | v29,23.4 v29,25.2 | v29,45.7 24.7,45.7 20.34,50.06 MOD1.D12 | v32,41.6 29.8,43.8 v29,43.8
MOSI  (via drill 0.25)
  Top 0.152: v32.4,46 33.2,45.2 v33.2,28.6 | v39.6,24.7 39.6,28.64 U2.4 | v35.6,26.8 37.2,25.2 v37.2,24.7
  Bottom 0.152: MOD1.D11 22.88,50.32 24.2,49 26.5,49 27.6,47.9 30.5,47.9 v32.4,46 | v37.2,24.7 v39.6,24.7 | v33.2,28.6 33.8,28.6 v35.6,26.8
N$1  (via drill 0.25)
  Top 0.203: v55.37,28.07 56.39,28.07 U4.19 | v53.85,29.59 51.82,29.59 51.56,29.84 U2.14
  Bottom 0.203: v53.85,29.59 v55.37,28.07
N$2  (via drill 0.25)
  Top 0.152: VOL.2 VOL.1 26.24,20.3 R11.1 20.36,19.3 v18.5,19.3 | C2.1 10.61,19.3 v14.3,19.3
  Bottom 0.152: v14.3,19.3 v18.5,19.3
N$3
  Top 0.203: C2.2 8.51,2.03 8.51,10.29 6.86,11.94 SP1.+
N$4  (via drill 0.25)
  Top 0.203: v55.37,26.04 56.39,26.04 U4.23 | v53.09,28.32 51.82,28.32 51.56,28.57 U2.13
  Bottom 0.203: v53.09,28.32 v55.37,26.04
N$6
  Top 0.203: U4.21 56.39,27.05 51.82,27.05 51.56,27.3 U2.12
N$7  (via drill 0.25)
  Top 0.203: v54.99,25.15 55.12,25.02 56.39,25.02 U4.25 | v53.72,25.15 52.7,25.15 51.82,26.04 51.56,26.04 U2.11
  Bottom 0.203: v53.72,25.15 v54.99,25.15
N$11
  Top 0.203: U3.8 49.4,20.57 53.34,16.64 L1.2
N$12
  Top 0.152: LED1.C 59.14,2.8 R10.2
N$13  (via drill 0.25)
  Top 0.203: v56.52,22.86 56.52,23.5 U4.28 | v56.77,21.08 57.4,21.08 57.66,20.83 C7.1
  Bottom 0.203: v56.52,22.86 56.52,21.34 v56.77,21.08
N$14
  Top 0.203: U5.4 55.88,10.67 55.88,11.3 55.12,12.06 55.12,12.83 55.37,13.08 61.21,13.08 61.34,12.95 61.34,10.54 60.83,10.03 C10.1
N$18  (via drill 0.25)
  Top 0.152: J1.2 62.66,46.49 v62.66,44.68 | v62.66,42.75 60.21,40.3 U4.8
  Bottom 0.152: v62.66,44.68 v62.66,42.75
N$19
  Top 0.152: J1.3 61.76,43.7 59.71,41.65 U4.9
N$30
  Top 0.152: J2.3 70.8,6.17 70.8,9.9 69.2,11.5 66.2,11.5 63.7,14 63.7,15.8 60.55,18.95 60.55,21.72 60.22,22.05 60.22,22.68 U4.35
N$31
  Top 0.152: U4.34 59.71,21.99 60.2,21.5 60.2,18.7 63.2,15.7 63.2,13.7 67.2,9.7 J2.2
NC
  Top 0.203: MOD1.NC 16.64,2.54 16.64,19.81 21.08,24.26 21.08,29.21 S1.A8
NOTCH_6050  (via drill 0.25)
  Top 0.152: SW1.5 22.9,5.1 31.4,5.1 32.8,6.5 R8.1 32.87,5.23 v32.9,5.2
  Bottom 0.152: MOD1.A3 44.97,0.5 36.1,0.5 35.7,0.9 35.7,3.9 34.4,5.2 v32.9,5.2
NOTCH_EN  (via drill 0.25)
  Top 0.152: SW1.4 v22.74,7.8 | v28.2,7.8 31.5,7.8 32.8,9.1 R7.1 34.17,7.8 36.6,7.8 38,6.4 38,5.4 38.9,4.5 42.51,4.5 MOD1.A2
  Bottom 0.152: v28.2,7.8 v22.74,7.8
PRESDA
  Top 0.203: R3.2 15.62,22.1 13.72,22.1 12.83,22.99 U1.5
SCL  (via drill 0.25)
  Top 0.152: R1.2 4,25 4,24.8 v3.2,24 | v7.9,21.9 8.39,22.39 U1.4
  Bottom 0.152: v7.9,21.9 6.1,20.1 1.8,20.1 0.8,21.1 0.8,24 2,24 | MOD1.SCL 4.4,47.56 4.4,40.4 2,38 2,24 | v3.2,24 2,24
SCLK  (via drill 0.25)
  Top 0.152: U2.5 40.3,27.36 v40.3,27.4 | v36.7,39.6 v35,39.6 | v21.5,42.5 21.9,42.1 30.3,42.1 v30.3,40 | v20.2,44.5 20.2,45.2 v19.3,46.1 | v17.2,46.4 17.2,50.2 MOD1.D13
  Bottom 0.152: v40.3,27.4 40.6,27.7 40.6,32.4 39,34 39,37.7 37.1,39.6 v36.7,39.6 | v35,39.6 30.7,39.6 v30.3,40 | v21.5,42.5 20.2,43.8 v20.2,44.5 | v19.3,46.1 17.5,46.1 v17.2,46.4
SDA  (via drill 0.25)
  Top 0.152: v27.2,26.9 v27.2,25.3 | v20.2,25 R2.2 R3.1
  Top 0.203: 17.14,21.97 17.4,21.97 R3.1 | 10.16,50.8 MOD1.SDA
  Bottom 0.152: v27.2,26.9 26.4,27.7 24,27.7 24,29.8 10.18,43.62 MOD1.SDA | v27.2,25.3 20.5,25.3 v20.2,25
SS  (via drill 0.25)
  Top 0.152: U2.3 v43.4,29.9 | v37,48.5 v35,48.5
  Bottom 0.152: v43.4,29.9 43.4,34.8 37.6,40.6 37.6,48.3 37.4,48.5 v37,48.5 | v35,48.5 27.72,48.5 MOD1.D10
VIN  (via drill 0.25)
  Top 0.152: v16.2,26.7 16.11,26.79 S1.A6
  Bottom 0.152: MOD1.VIN 31.75,5.1 24.3,5.1 19.7,9.7 19.7,23.2 v16.2,26.7

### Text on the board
tNames: IN0 | Intan Technologies | intantech.com | B | 1 | 8 | A | IN15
